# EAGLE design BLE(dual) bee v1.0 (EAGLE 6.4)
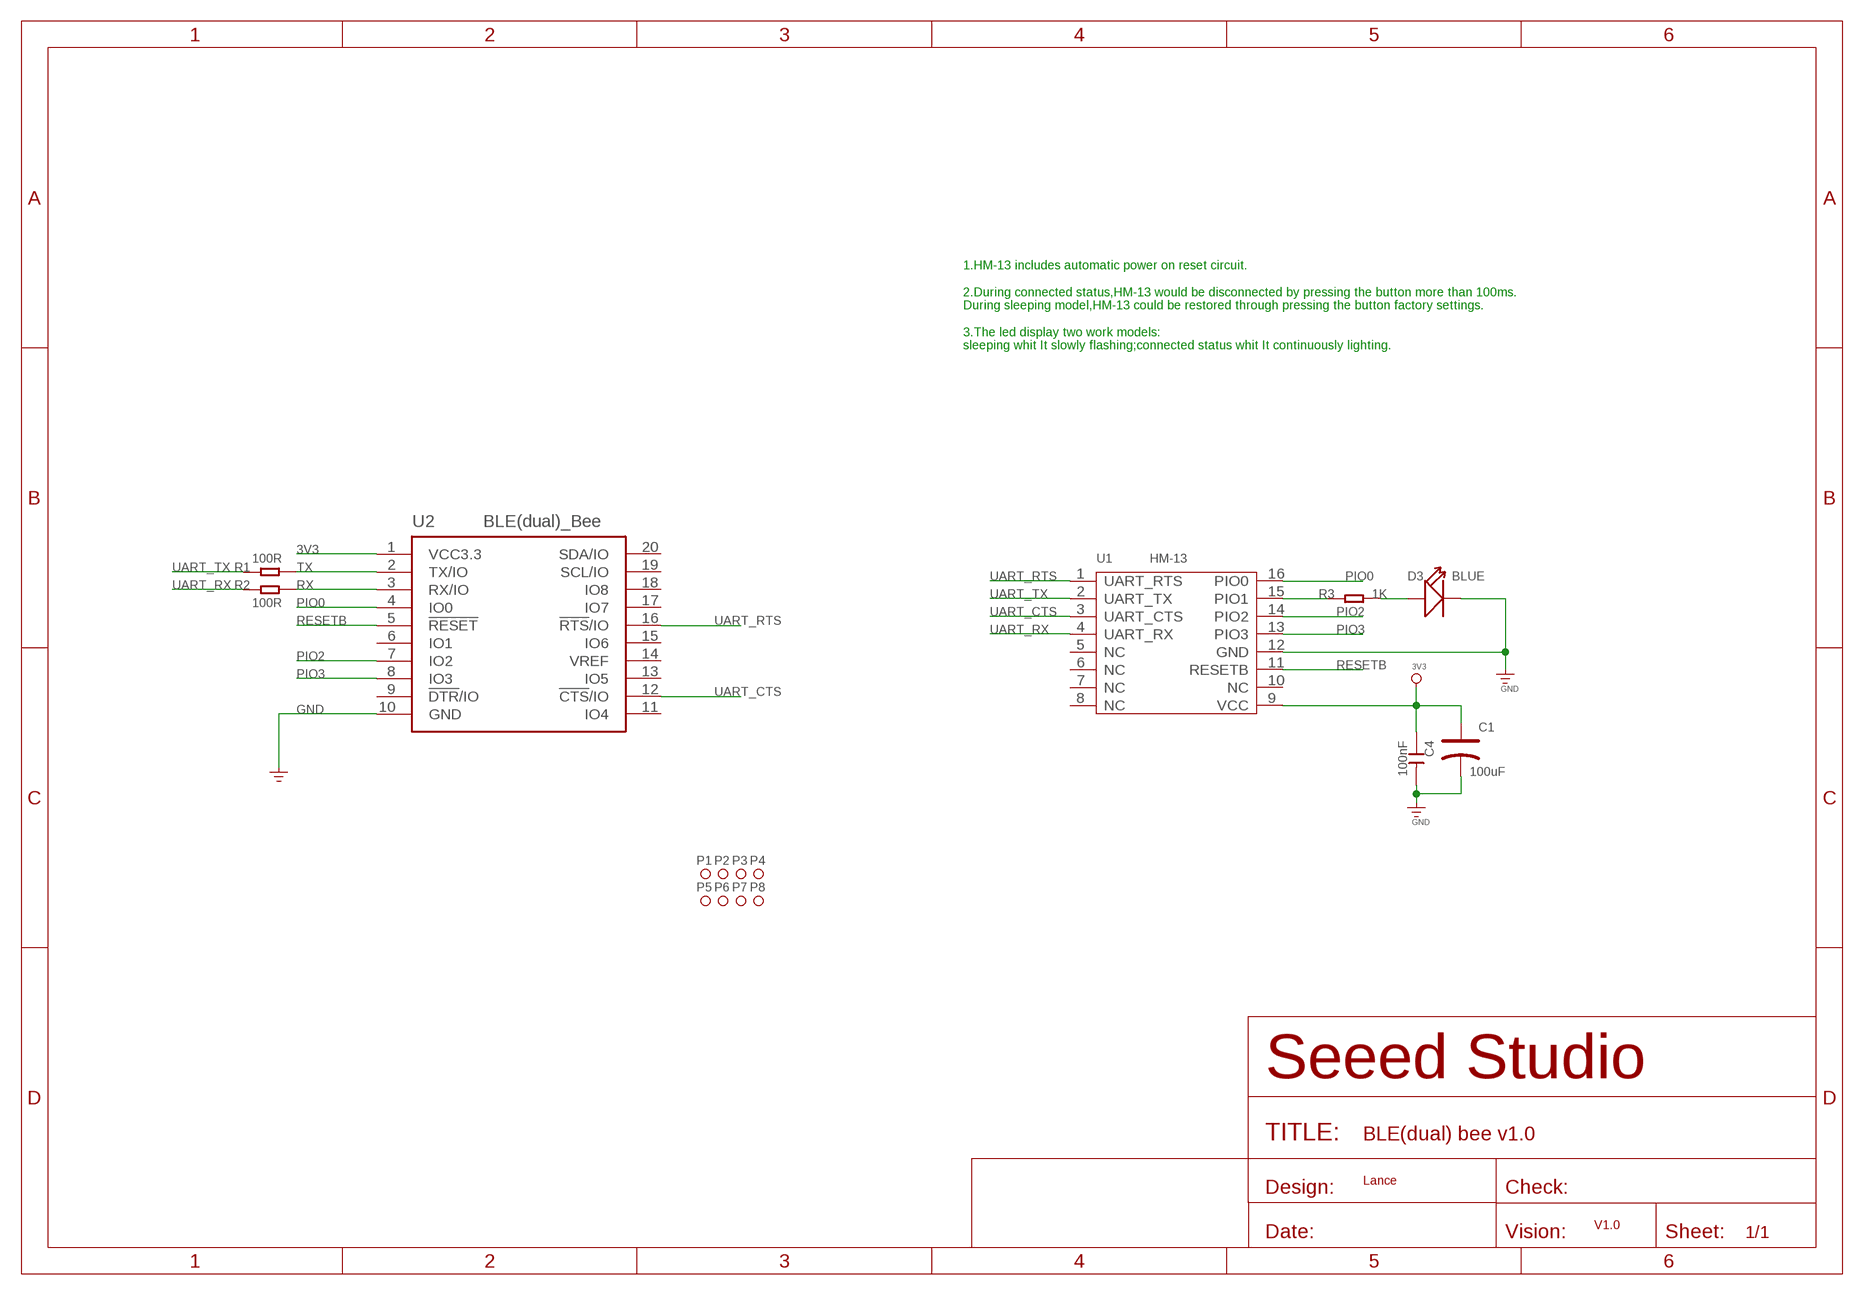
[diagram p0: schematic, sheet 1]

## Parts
C1  100uF  CAP-POLAR-AVX-B  [AVX-B]
C4  100nF  C-0603  [C0603]
D3  BLUE  LED'0603'  [LED-0603]
P1  PAD-MARK'ANNULAR'  [ROUND-MARK-1.0]
P2  PAD-MARK'ANNULAR'  [ROUND-MARK-1.0]
P3  PAD-MARK'ANNULAR'  [ROUND-MARK-1.0]
P4  PAD-MARK'ANNULAR'  [ROUND-MARK-1.0]
P5  PAD-MARK'ANNULAR'  [ROUND-MARK-1.0]
P6  PAD-MARK'ANNULAR'  [ROUND-MARK-1.0]
P7  PAD-MARK'ANNULAR'  [ROUND-MARK-1.0]
P8  PAD-MARK'ANNULAR'  [ROUND-MARK-1.0]
R1  100R  R-0603  [R0603]
R2  100R  R-0603  [R0603]
R3  1K  R-0603  [R0603]
U1  HM-13  MOUDLE-BLUETOOTH-HM-13  [16P-L18.5*W13.5*H2.3MM]
U2  BLE(dual)_Bee  BEE-2X10P-2.0'DIM'  [BEE-2X10P-DIP-2.0-DIM]

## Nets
3V3: C1.+ C4.1 U1.9(VCC) U2.1(VCC3.3)
GND: C1.- C4.2 D3.- U1.12(GND) U2.10(GND) ; supply symbol labelled GND_POWER
N$7: R3.1 U1.15(PIO1)
N$8: D3.+ R3.2
PIO0: U1.16(PIO0) U2.4(IO0)
PIO2: U1.14(PIO2) U2.7(IO2)
PIO3: U1.13(PIO3) U2.8(IO3)
RESETB: U1.11(RESETB) U2.5(!RESET)
RX: R2.2 U2.3(RX/IO)
TX: R1.2 U2.2(TX/IO)
UART_CTS: U1.3(UART_CTS) U2.12(!CTS!/IO)
UART_RTS: U1.1(UART_RTS) U2.16(!RTS!/IO)
UART_RX: R2.1 U1.4(UART_RX)
UART_TX: R1.1 U1.2(UART_TX)
Unconnected: U1.5(NC) U1.6(NC) U1.7(NC) U1.8(NC) U1.10(NC) U2.6(IO1) U2.9(!DTR!/IO) U2.11(IO4) U2.13(IO5) U2.14(VREF) U2.15(IO6) U2.17(IO7) U2.18(IO8) U2.19(SCL/IO) U2.20(SDA/IO)

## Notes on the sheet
- 1.HM-13 includes automatic power on reset circuit.
   
  2.During connected status,HM-13 would be disconnected by pressing the button more than 100ms.
  During sleeping model,HM-13 could be restored through pressing the button factory settings.
  
  3.The led display two work models:
  sleeping whit It slowly flashing;connected status whit It continuously lighting.
- Lance
- V1.0

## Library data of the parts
C1 = Discrete-new:CAP-POLAR: Electrolytic Capacitors,Tantalum Capacitors and Super Capacitors
C4 = Discrete:C*: Ceramic Capacitors
D3 = Discrete-new:LED
P1-P8 = Discrete-new:PAD-MARK; PARTNO: DNP
R1-R3 = Discrete:R*
U1 = template:MOUDLE-BLUETOOTH-HM-13: Bluetooth Specification V4.0 EDR and BLE
U2 = moudle-new:BEE-2X10P-2.0

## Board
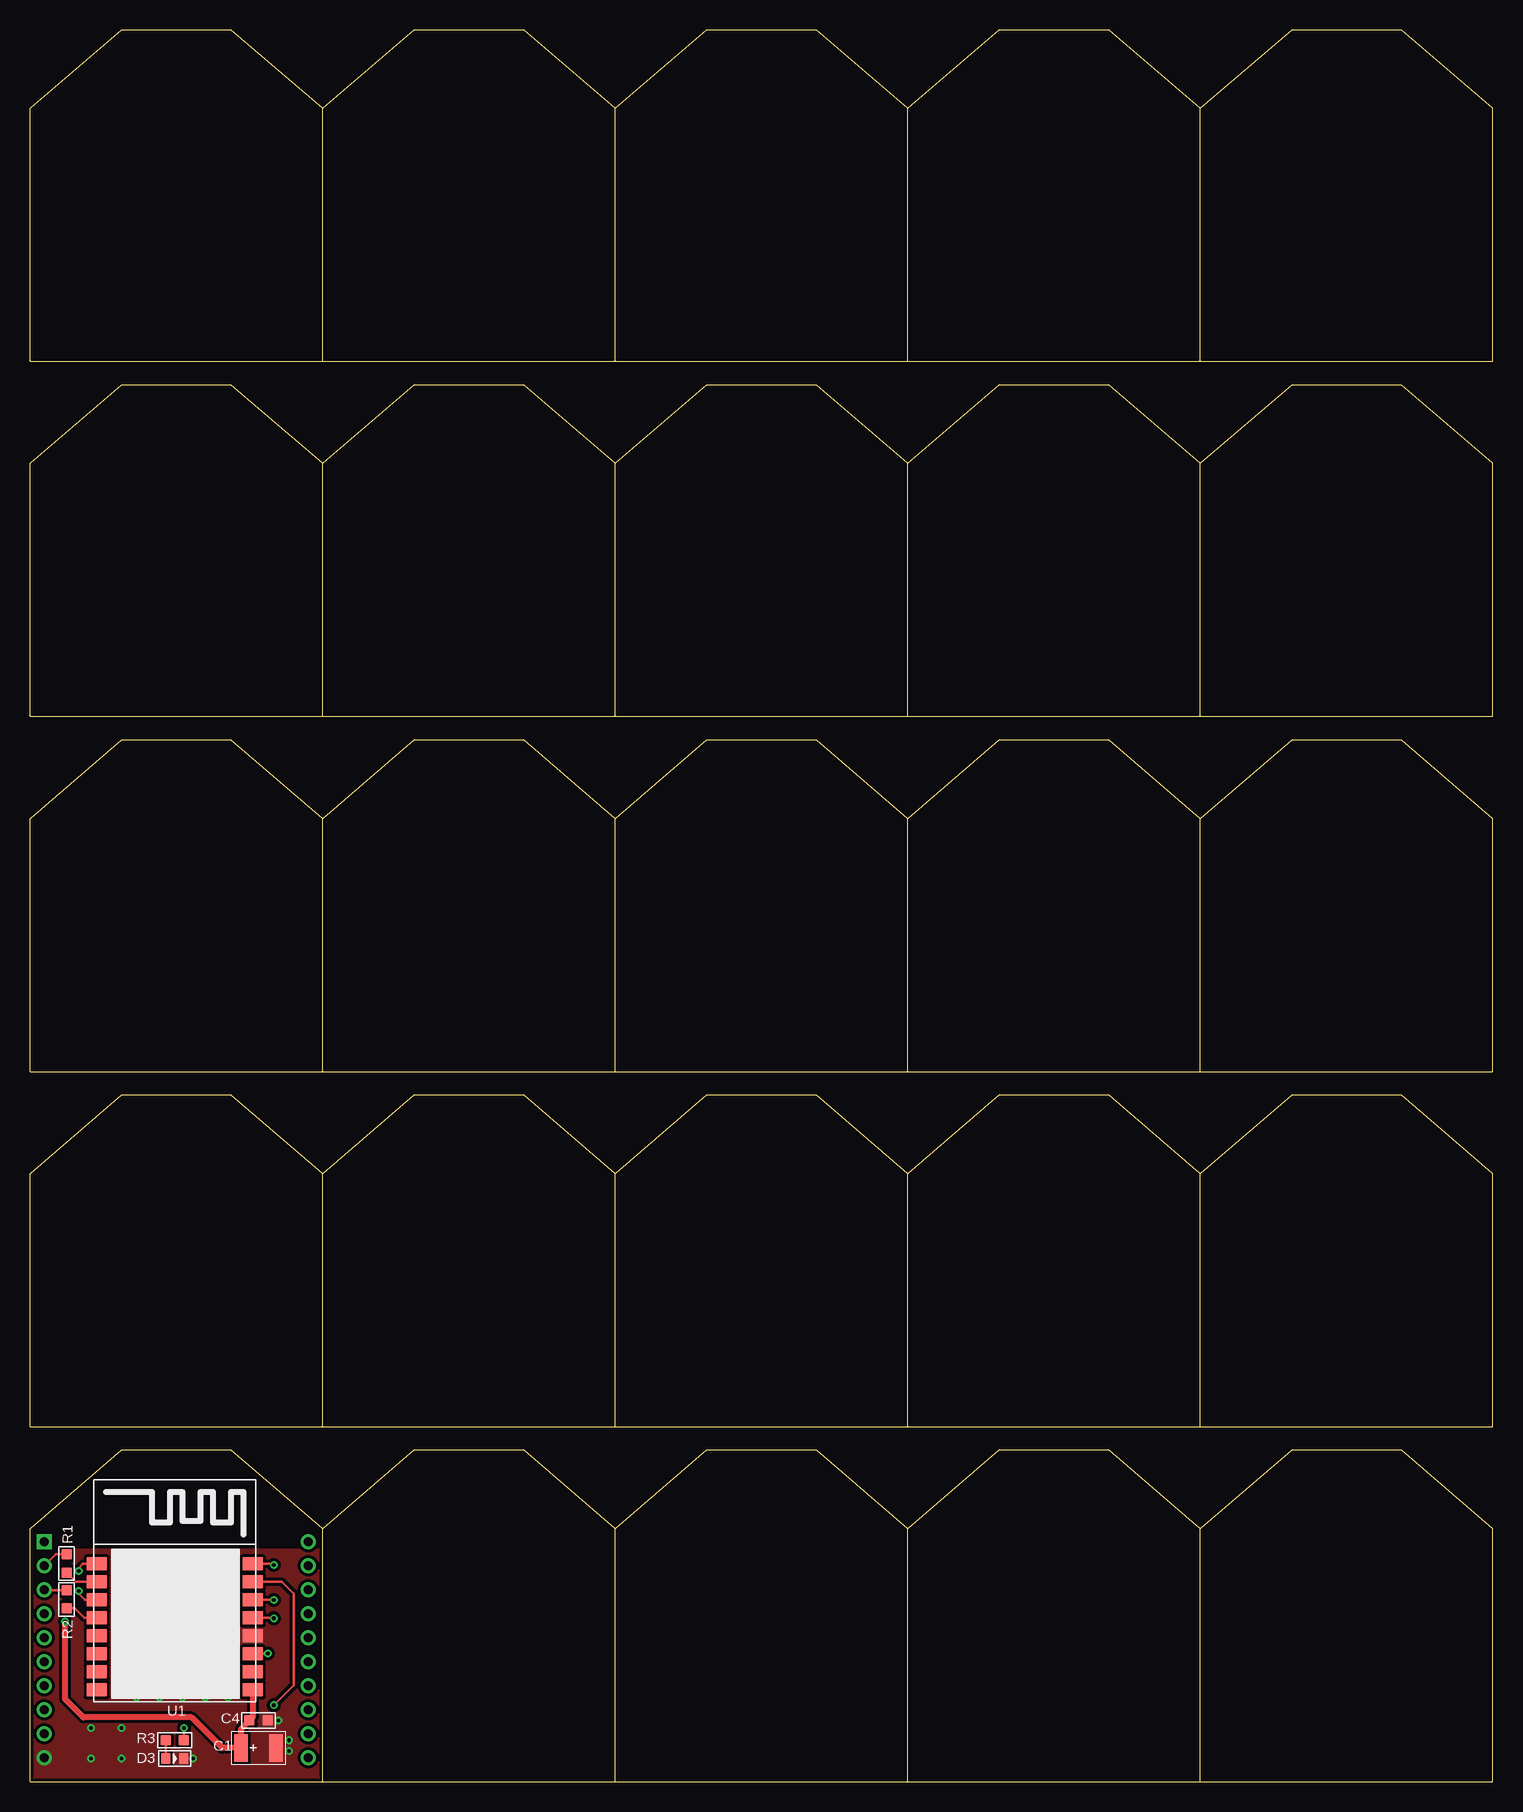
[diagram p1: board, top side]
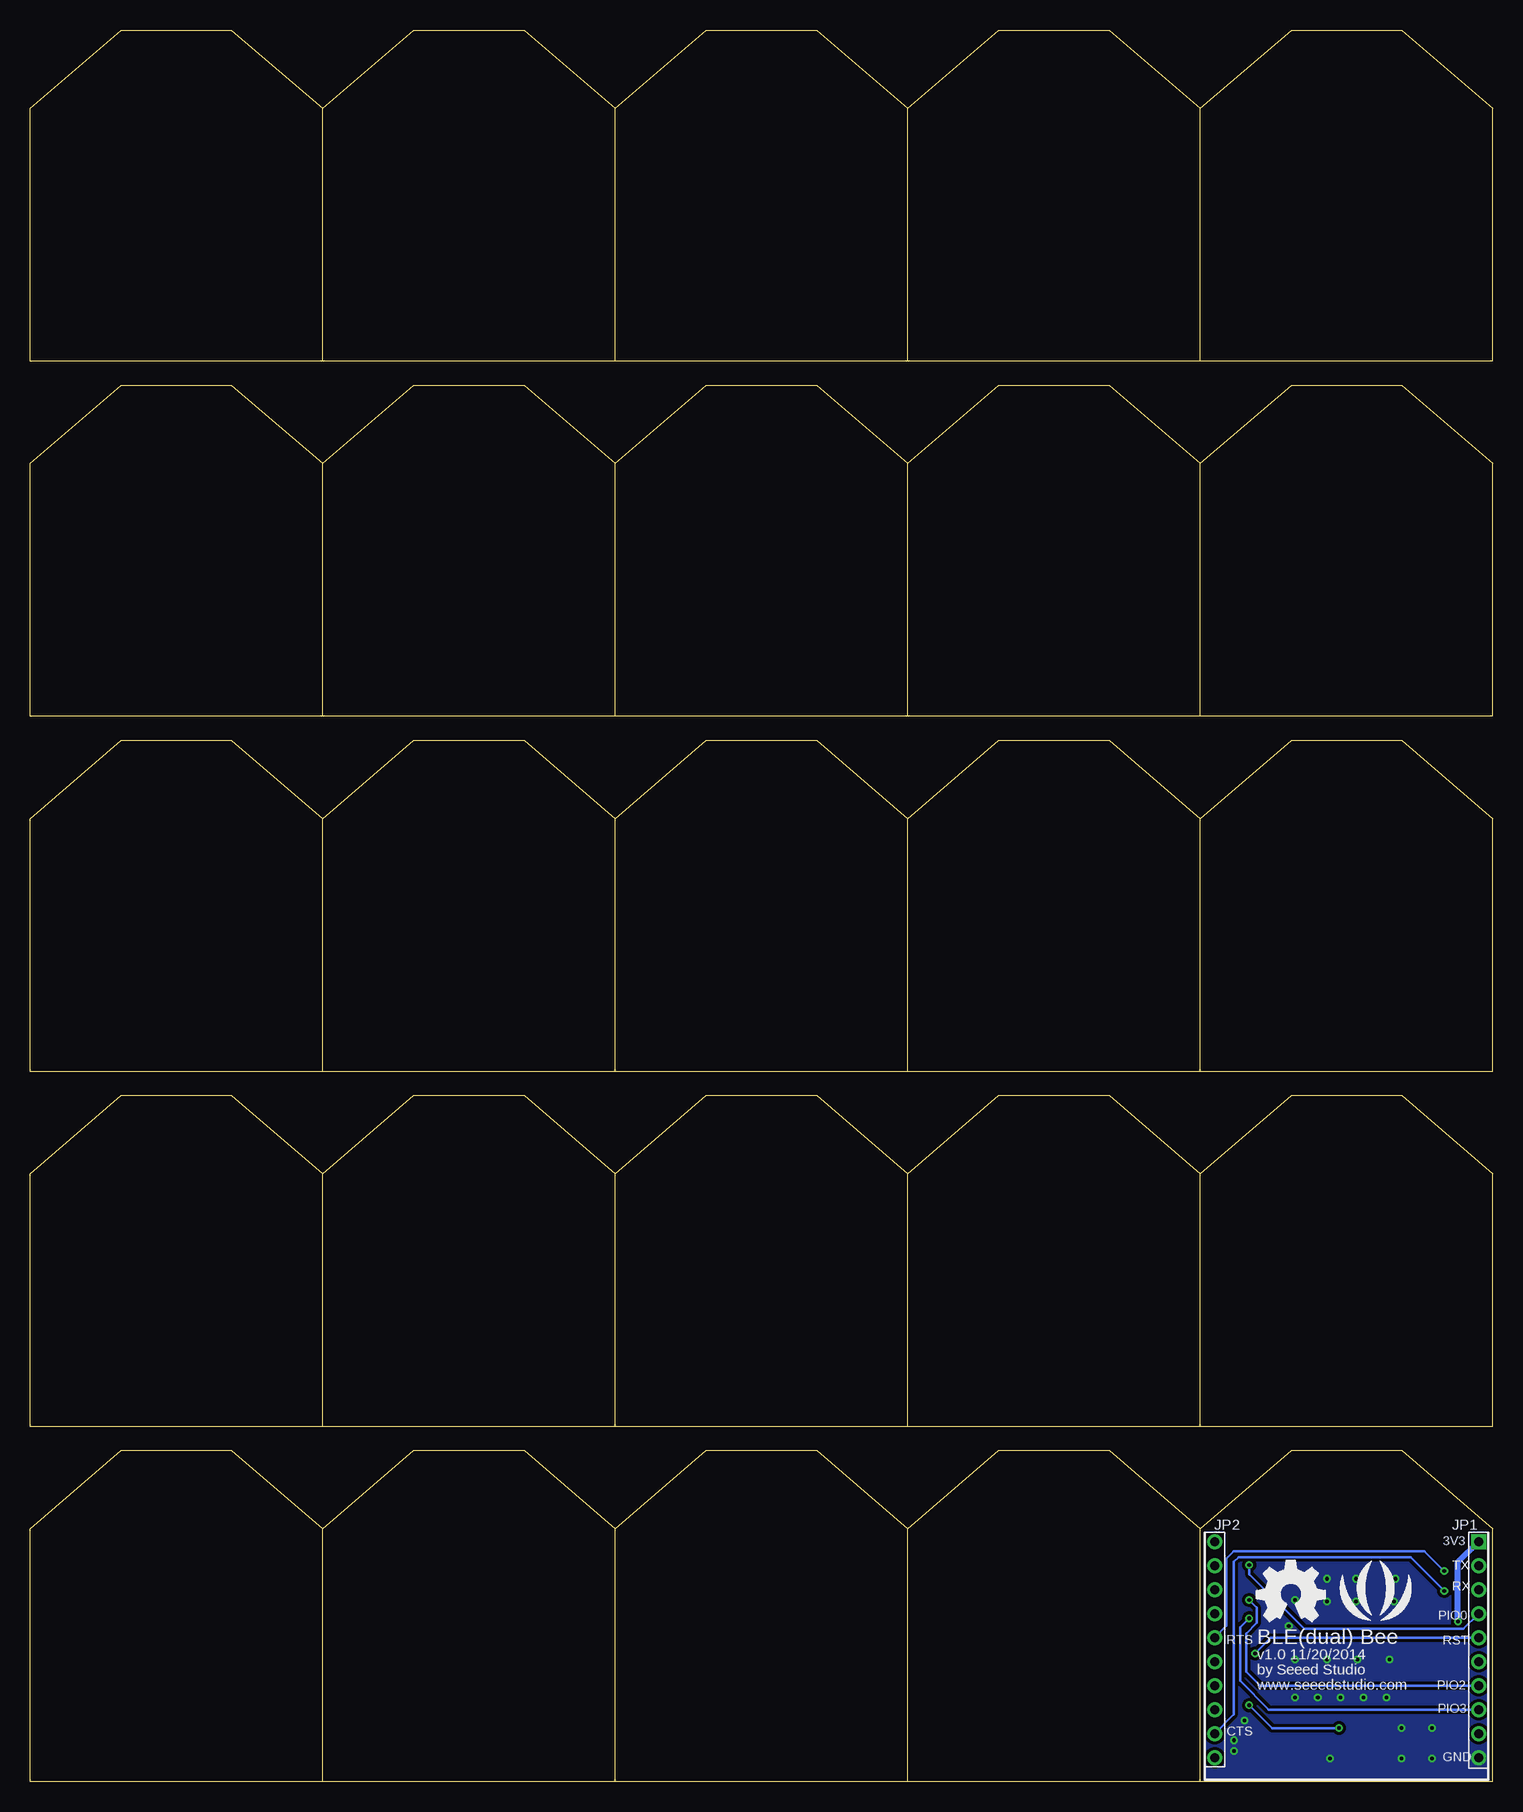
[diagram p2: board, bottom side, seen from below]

Size 121.92 x 145.97 mm. Coordinates in mm from the lower left corner, seen from the top.
Copper layers (1*16): Top 0.035mm / dielectric 1.5mm / Bottom 0.035mm
Design rules "SeeedStudio_2layer_DRU_no_angle_20140221 *": minimum track width 6mil, minimum drill 12mil, track to track 6mil, track to pad 6mil, pad to pad 6mil, via to via 6mil, smd to smd 0mil, copper to edge 10mil, drill to drill 10mil, minimum pad ring 10mil, minimum via ring 6mil, stop-mask expansion 2mil, vias tented up to drill 25mil, thermal gap 10mil
Holes 2.03 mm at -4.45,143.54 -4.45,2.57 126.36,143.54 126.36,2.57
tRestrict: area -0.3,19.7 to 25.3,27.7
bRestrict: area -0.3,19.7 to 25.3,27.7

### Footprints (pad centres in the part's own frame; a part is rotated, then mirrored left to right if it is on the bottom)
AVX-B = smd 1.143 x 2.286: + -1.46,0; - 1.46,0
C0603 = smd 0.889 x 0.889: 1 -0.762,0; 2 0.762,0
LED-0603 = smd 0.762 x 0.889: + -0.762,0; - 0.762,0
ROUND-MARK-1.0 = smd 1.016 x 1.016: P$1 0,0
R0603 = smd 0.889 x 0.889: 1 -0.762,0; 2 0.762,0
16P-L18.5*W13.5*H2.3MM = smd 1.7 x 1.1: 1 -6.5,2.25; 2 -6.5,0.75; 3 -6.5,-0.75; 4 -6.5,-2.25; 5 -6.5,-3.75; 6 -6.5,-5.25; 7 -6.5,-6.75; 8 -6.5,-8.25; 9 6.5,-8.25; 10 6.5,-6.75; 11 6.5,-5.25; 12 6.5,-3.75; 13 6.5,-2.25; 14 6.5,-0.75; 15 6.5,0.75; 16 6.5,2.25
BEE-2X10P-DIP-2.0-DIM = drill 0.762 pad 1.27 square: 1 -11,6.195 | drill 0.762 pad 1.27: 2 -11,4.195; 3 -11,2.195; 4 -11,0.195; 5 -11,-1.805; 6 -11,-3.805; 7 -11,-5.805; 8 -11,-7.805; 9 -11,-9.805; 10 -11,-11.805; 11 11,-11.805; 12 11,-9.805; 13 11,-7.805; 14 11,-5.805; 15 11,-3.805; 16 11,-1.805; 17 11,0.195; 18 11,2.195; 19 11,4.195; 20 11,6.195

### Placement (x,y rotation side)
C1  19.05,2.82 0 top
C4  19.05,5.11 0 top
D3  12.06,1.93 0 top
P1  not placed on the board
P2  not placed on the board
P3  not placed on the board
P4  not placed on the board
P5  not placed on the board
P6  not placed on the board
P7  not placed on the board
P8  not placed on the board
R1  3.05,18.19 90 top
R2  3.05,15.2 90 top
R3  12.06,3.45 180 top
U1  12.06,15.9 0 top
U2  12.19,13.8 0 top
U3  [BEE-2X10P-DIP-2.0-DIM']  12.19,72.99 0 top
U4  [BEE-2X10P-DIP-2.0-DIM']  12.19,102.58 0 top
U5  [BEE-2X10P-DIP-2.0-DIM']  12.19,132.17 0 top
U6  [BEE-2X10P-DIP-2.0-DIM']  36.57,43.4 0 top
U7  [BEE-2X10P-DIP-2.0-DIM']  36.57,72.99 0 top
U8  [BEE-2X10P-DIP-2.0-DIM']  12.19,43.4 0 top
U9  [BEE-2X10P-DIP-2.0-DIM']  36.57,102.58 0 top
U10  [BEE-2X10P-DIP-2.0-DIM']  36.57,132.17 0 top
U11  [BEE-2X10P-DIP-2.0-DIM']  60.96,102.58 0 top
U12  [BEE-2X10P-DIP-2.0-DIM']  60.96,132.17 0 top
U13  [BEE-2X10P-DIP-2.0-DIM']  85.34,102.58 0 top
U14  [BEE-2X10P-DIP-2.0-DIM']  85.34,132.17 0 top
U15  [BEE-2X10P-DIP-2.0-DIM']  60.96,43.4 0 top
U16  [BEE-2X10P-DIP-2.0-DIM']  60.96,72.99 0 top
U17  [BEE-2X10P-DIP-2.0-DIM']  85.34,43.4 0 top
U18  [BEE-2X10P-DIP-2.0-DIM']  85.34,72.99 0 top
U19  [BEE-2X10P-DIP-2.0-DIM']  36.57,13.8 0 top
U20  [BEE-2X10P-DIP-2.0-DIM']  60.96,13.8 0 top
U21  [BEE-2X10P-DIP-2.0-DIM']  85.34,13.8 0 top
U22  [BEE-2X10P-DIP-2.0-DIM']  109.73,102.58 0 top
U23  [BEE-2X10P-DIP-2.0-DIM']  109.73,132.17 0 top
U24  [BEE-2X10P-DIP-2.0-DIM']  109.73,43.4 0 top
U25  [BEE-2X10P-DIP-2.0-DIM']  109.73,72.99 0 top
U26  [BEE-2X10P-DIP-2.0-DIM']  109.73,13.8 0 top
U$1  [OSHW_FILLX200_NOTEXT]  19.68,13.36 0 bottom
U$6  [SEEED-SILK-280*268MIL]  9.78,15.14 0 bottom

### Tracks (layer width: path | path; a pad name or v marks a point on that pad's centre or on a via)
3V3  (via drill 0.3 pad 0.64)
  Top 0.508: U1.9 18.56,5.38 C4.1 17.59,4.41 C1.+ 16,2.82 13.46,5.36 4.44,5.36 2.92,6.88 v2.92,13.36
  Bottom 0.508: v2.92,13.36 2.92,18.27 U2.1
GND  (via drill 0.3 pad 0.64)
  other vias: 13.59,1.93 21.59,2.57 21.59,3.45 20.7,5.11 8.89,7.01 10.79,7.01 12.7,7.01 16.51,7.01 14.6,7.01 8.13,16.92 8.25,15.01 8.63,10.19 11.3,10.19 13.84,10.19 16.51,10.19 16.51,15.14 13.84,15.01 11.43,15.01 13.84,16.92 11.43,16.92 17.02,12.98 7.62,1.93 7.62,4.47 5.08,4.47 5.08,1.93
  pour Top (isolate 0.254, rank 6, no thermals): -1.27,28.6 25.4,28.6 25.4,-1.24 -1.27,-1.24
  pour Bottom (isolate 0.254, rank 6, no thermals): -1.27,28.6 25.4,28.6 25.4,-1.24 -1.27,-1.24
N$7  (via drill 0.3 pad 0.64)
  Top 0.203: R3.1 v12.82,4.47 | U1.15 20.96,16.65 21.97,15.65 21.97,8.03 v20.32,6.38
  Bottom 0.203: v20.32,6.38 18.41,4.47 v12.82,4.47
N$8
  Top 0.203: D3.+ R3.2
PIO0  (via drill 0.3 pad 0.64)
  Top 0.203: U1.16 20.23,18.15 v20.32,18.06
  Bottom 0.203: U2.4 2.46,12.73 15.75,12.73 20.32,17.3 v20.32,18.06
PIO2  (via drill 0.3 pad 0.64)
  Top 0.203: U1.14 20.31,15.15 v20.32,15.14
  Bottom 0.203: U2.7 19.4,8 20.57,9.17 20.57,12.34 19.68,13.23 19.68,14.5 v20.32,15.14
PIO3  (via drill 0.3 pad 0.64)
  Top 0.203: U1.13 20.28,13.65 v20.32,13.61
  Bottom 0.203: U2.8 18.67,6 21.08,8.41 21.08,12.85 v20.32,13.61
RESETB  (via drill 0.3 pad 0.64)
  Top 0.203: U1.11 19.77,10.65 v19.81,10.69
  Bottom 0.203: U2.5 18.5,12 v19.81,10.69
RX
  Top 0.203: R2.2 1.23,15.96 U2.3
TX
  Top 0.203: R1.2 2.14,18.95 U2.2
UART_CTS  (via drill 0.3 pad 0.64)
  Top 0.203: U1.3 4.56,15.15 4.06,15.65 v4.06,15.9
  Bottom 0.203: U2.12 23.19,4.01 21.59,5.61 21.59,18.31 21.21,18.69 6.86,18.69 v4.06,15.9
UART_RTS  (via drill 0.3 pad 0.64)
  Top 0.203: U1.1 4.41,18.15 4.06,17.81 v4.06,17.55
  Bottom 0.203: U2.16 23.19,12.01 22.22,12.98 22.22,18.57 21.59,19.2 5.71,19.2 v4.06,17.55
UART_RX
  Top 0.203: R2.1 3.74,14.44 4.53,13.65 U1.4
UART_TX
  Top 0.203: U1.2 3.82,16.65 R1.1

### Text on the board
bPlace: JP1 | JP2 | 3V3 | TX | RX | PIO0 | RST | BLE(dual) Bee | RTS | v1.0 11/20/2014 | by Seeed Studio | PIO2 | www.seeedstudio.com | PIO3 | CTS | GND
